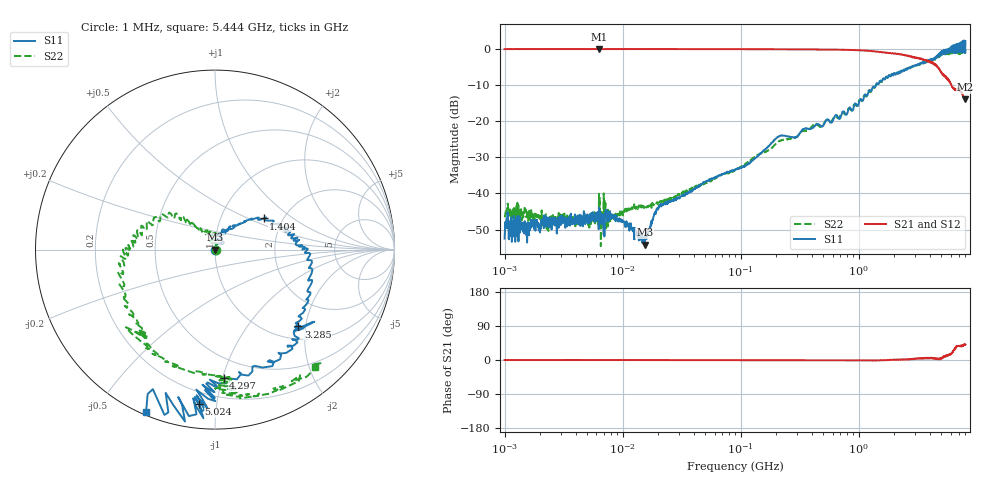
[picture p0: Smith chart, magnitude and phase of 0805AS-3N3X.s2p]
!s-Parameter Generated by FASTRON Sdn. Bhd.
!FASTRON P/N : 0805AS-3N3X
!Keysight Technologies: E5071C_MY46733604_B.14.02
!Date: Mon Jun 15 12:46:31 2026
!Version  :Rev01  Mon Jun 15 12:46:31 2026
!Data & Calibration Information:
!Freq  S11:SOLT2(ON)  S21:SOLT2(ON)  S12:SOLT2(ON)  S22:SOLT2(ON)
!PortZ  Port1:50+j0  Port2:50+j0
!When reading reference impedance value at option line is always used.
! Remarks : This data is being provided solely for informational purposes.
# Hz S dB R 50
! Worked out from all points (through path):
!   1601 points, 1 MHz to 8 GHz, reference 50 ohm
!   highest |S21| = 0.01 dB at 6.301 MHz (marker M1); lowest = -13.9 dB at 7.923 GHz (marker M2)
!   lowest |S11| = -54.2 dB at 15.35 MHz (marker M3), VSWR 1.00, Z = 50.2 + j0.0175 ohm
!   |S11| at or under -10 dB: start of sweep to 1.399 GHz
!   |S22| runs from -54.6 to -0.2 dB; largest |S21 - S12| = 0.0084
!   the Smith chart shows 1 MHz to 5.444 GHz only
!   S11 on the Smith chart (normalised r, x): 1 MHz: 1.00, -0.00; 1.404 GHz: 1.59, +0.62; 3.285 GHz: 1.28, -1.82; 4.297 GHz: 0.34, -1.01; 5.024 GHz: 0.13, -0.89; 5.444 GHz: 0.01, -0.66
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1000000  -52.50 -10.7  -0.05 -0.1  -0.04 -0.1  -46.20 4.2
4479405  -47.50 5.1  -0.05 -0.0  -0.05 -0.1  -47.90 12.1
6301378  -44.00 18.7  0.01 -0.3  -0.01 0.0  -40.10 30.9
1.535471e7  -54.20 5.1  -0.04 -0.1  -0.06 -0.1  -43.40 25.6
2.00676e7  -43.90 36.2  -0.05 -0.1  -0.06 -0.1  -42.70 47.6
8.994653e7  -33.40 72.5  -0.06 -0.3  -0.07 -0.3  -33.50 70.4
2.111884e8  -24.20 37.9  -0.11 -0.3  -0.12 -0.3  -25.60 129.0
4.006501e8  -22.00 93.5  -0.15 -0.4  -0.16 -0.4  -21.50 80.4
7.765934e8  -18.20 60.4  -0.25 -0.6  -0.26 -0.6  -18.10 125.0
1.403687e9  -9.86 32.7  -0.78 -1.2  -0.79 -1.3  -9.77 141.0
1.7949e9  -7.41 14.1  -1.20 0.1  -1.20 -0.1  -7.32 162.0
2.486897e9  -5.58 -2.1  -1.82 2.0  -1.87 1.7  -5.56 -176.0
3.284549e9  -3.99 -42.7  -2.60 4.8  -2.62 4.9  -4.34 -131.0
3.730463e9  -3.62 -49.3  -3.30 4.3  -3.30 4.4  -3.55 -123.0
4.296652e9  -2.90 -86.2  -4.03 3.5  -4.02 2.9  -3.03 -87.3
5.02444e9  -1.24 -95.9  -6.67 5.9  -6.70 5.3  -1.70 -80.4
5.444317e9  -0.14 -113.0  -7.49 11.0  -7.55 10.6  -1.31 -49.7
6.110812e9  0.17 -128.0  -10.20 18.5  -10.20 17.5  -1.22 -29.4
6.534915e9  1.16 -124.0  -11.20 31.6  -11.20 30.6  -0.53 4.4
6.959019e9  -0.73 -145.0  -11.30 37.2  -11.20 36.5  -0.94 43.4
7.92289e9  1.42 -166.0  -13.90 41.1  -13.60 40.5  -0.18 75.8
8e9  2.21 -179.0  -13.80 40.8  -13.60 40.5  -0.29 72.9
